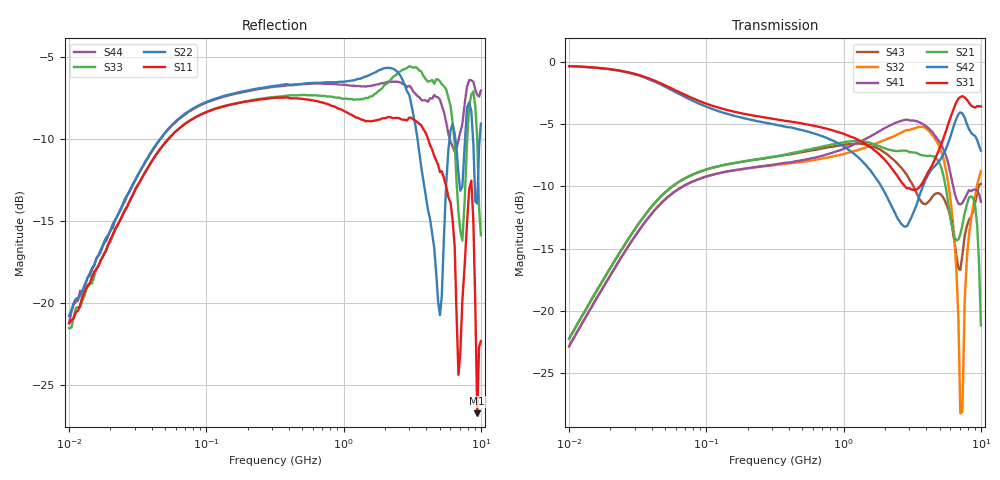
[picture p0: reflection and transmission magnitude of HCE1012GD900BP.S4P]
!Agilent Technologies,E5071C,MY46111244,A.11.31
!Date: Tue May 14 17:33:55 2019
!Data & Calibration Information:
!Freq	S11:SOLT4(ON)	S12:SOLT4(ON)	S13:SOLT4(ON)	S14:SOLT4(ON)
!	S21:SOLT4(ON)	S22:SOLT4(ON)	S23:SOLT4(ON)	S24:SOLT4(ON)
!	S31:SOLT4(ON)	S32:SOLT4(ON)	S33:SOLT4(ON)	S34:SOLT4(ON)
!	S41:SOLT4(ON)	S42:SOLT4(ON)	S43:SOLT4(ON)	S44:SOLT4(ON)
!PortZ  Port1:50+j0  Port2:50+j0  Port3:50+j0  Port4:50+j0
!Above PortZ is port z conversion or system Z0 setting when saving the data.
!When reading, reference impedance value at option line is always used.
# Hz S dB R 50
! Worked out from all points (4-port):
!   201 points, 10 MHz to 10 GHz, reference 50 ohm
!   strongest paths, dB at 10 MHz, 56.66 MHz, 319.3 MHz, 1.79 GHz, 10 GHz:
!     S31: -0.4, -2.2, -4.6, -7.4, -3.6
!     S42: -0.4, -2.3, -5.1, -9.6, -7.1
!     S21: -22.2, -10.0, -7.6, -6.7, -21.2
!     S41: -22.8, -10.6, -8.2, -5.6, -11.2
!     S32: -22.9, -10.5, -8.3, -6.5, -8.8
!     S43: -22.2, -10.0, -7.6, -7.0, -9.8
!   lowest |S11| = -26.7 dB at 9.406 GHz (marker M1), VSWR 1.10, Z = 50 + j4.61 ohm
!   |S11| at or under -10 dB: start of sweep to 52.73 MHz; 4.13 GHz to end of sweep
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1e7  -21.24 60.8  -22.24 80.6  -0.35 -4.8  -22.81 -100.0
     -22.24 80.7  -20.79 58.6  -22.85 -100.0  -0.37 -5.1
     -0.36 -4.7  -22.85 -99.9  -21.54 60.9  -22.23 80.4
     -22.85 -100.0  -0.36 -5.1  -22.24 80.4  -21.18 60.8
1.617948e9  -8.90 -19.1  -6.56 -10.3  -6.93 -77.8  -5.93 77.5
            -6.58 -10.5  -6.00 -19.8  -6.69 85.8  -8.91 -87.3
            -6.96 -78.1  -6.68 85.7  -7.38 -15.4  -6.77 -14.2
            -5.89 77.9  -8.93 -87.6  -6.77 -14.4  -6.72 -33.1
4.879977e9  -11.57 -89.3  -7.88 -42.8  -7.29 66.5  -6.24 -42.4
            -7.95 -42.9  -19.90 -99.4  -6.62 -49.9  -8.14 20.0
            -7.27 66.9  -6.61 -49.8  -6.36 -89.3  -10.48 -23.8
            -6.27 -43.0  -8.07 20.1  -10.55 -24.3  -7.44 -138.8
7.079458e9  -23.10 169.3  -13.86 -32.8  -2.81 -15.9  -11.65 -66.1
            -13.86 -33.3  -13.14 -81.3  -28.00 -106.2  -4.11 -41.1
            -2.84 -16.3  -28.22 -108.1  -15.57 -78.0  -16.63 -12.4
            -11.45 -66.7  -4.07 -41.8  -16.71 -12.0  -9.56 156.6
8.515692e9  -12.53 172.6  -10.68 -58.5  -3.57 -62.0  -10.19 -75.8
            -10.81 -57.9  -8.29 -178.7  -12.54 -27.2  -5.79 -80.3
            -3.55 -62.0  -12.45 -28.2  -7.29 -151.6  -12.52 -12.2
            -10.39 -75.4  -5.73 -80.5  -12.43 -11.2  -6.40 145.8
9.406277e9  -26.73 87.6  -13.07 -97.8  -3.62 -82.9  -10.30 -88.4
            -13.20 -97.6  -13.93 78.4  -9.98 -43.0  -6.26 -99.3
            -3.57 -83.1  -9.84 -42.7  -9.98 -158.3  -10.57 -20.0
            -10.34 -88.2  -6.31 -100.3  -10.51 -20.3  -7.31 118.0
1e10  -22.32 32.7  -21.64 -125.2  -3.59 -100.1  -11.28 -97.4
      -21.16 -125.5  -9.05 30.7  -8.81 -55.0  -7.19 -109.7
      -3.59 -100.2  -8.80 -54.5  -15.86 174.9  -9.78 -39.3
      -11.23 -97.5  -7.13 -110.7  -9.81 -39.5  -7.03 100.3
